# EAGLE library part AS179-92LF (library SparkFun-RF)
SKYWORKS SOLUTIONS - AS179-92LF - IC, SWITCH, RF, SPDT, 0.02-3.0GHZ Source: Datasheet
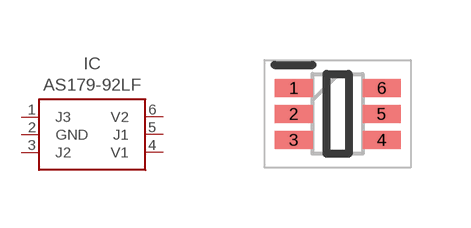
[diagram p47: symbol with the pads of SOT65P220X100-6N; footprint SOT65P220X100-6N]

Designator prefix IC

## AS179-92LF (PROD_ID: IC-15047)  [SOT65P220X100-6N]
1  J3
2  GND  pwr
3  J2
4  V1  pwr
5  J1
6  V2  pwr

## Footprint SOT65P220X100-6N (pad centres in mm)
AS179-92LF
smd 0.95 x 0.45: 1 -1.1,0.65; 2 -1.1,0; 3 -1.1,-0.65; 4 1.1,-0.65; 5 1.1,0; 6 1.1,0.65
